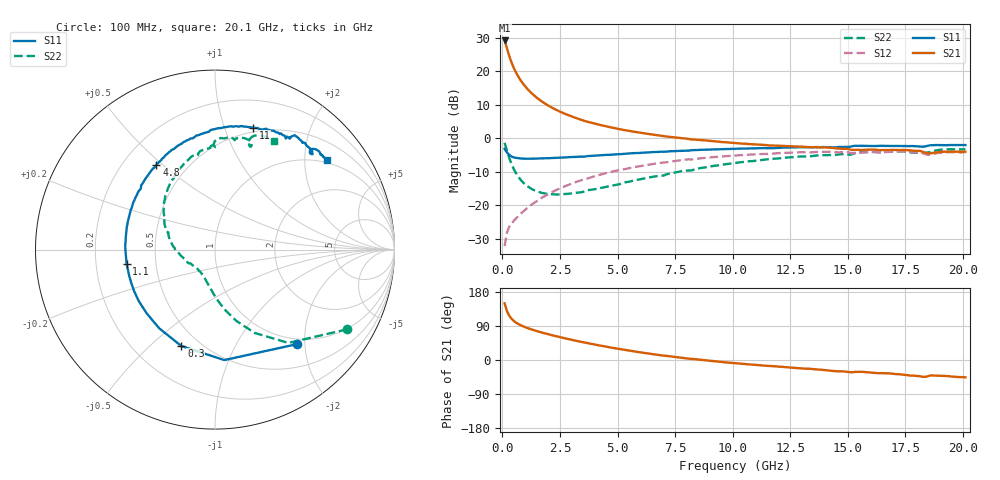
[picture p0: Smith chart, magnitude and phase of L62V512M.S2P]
!  Infineon Technologies AG
! BFR380L3 , PF131585-7, No.6, Th 09.10.01, soldered on pcb-board, measured with PP GSG850
!  Vce=2.5 V,  Ic=12.5 mA
! Common Emitter S-Parameters:  15. November 2001
#  GHz  S  MA  R  50
! f  S11  S21  S12  S22
! GHz  Mag  Ang  Mag  Ang  Mag  Ang  Mag  Ang
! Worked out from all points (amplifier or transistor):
!   201 points, 100 MHz to 20.1 GHz, reference 50 ohm
!   highest |S21| = 29.3 dB at 100 MHz (marker M1)
!   |S21| within 3 dB of that: start of sweep to 228.5 MHz
!   unconditionally stable (mu >= 1): 1.666 GHz to 4.494 GHz
!   at 3.4 GHz: K = 1.02, MAG = 8.1 dB, |S12| = -12.5 dB
!   at 10.1 GHz: K = 0.95, MSG = 1.9 dB, |S12| = -5.1 dB
!   at 20.1 GHz: K = 0.99, MSG = 0.1 dB, |S12| = -4.1 dB
!   S11 on the Smith chart (normalised r, x): 100 MHz: 0.90, -1.85; 300 MHz: 0.40, -0.63; 1.1 GHz: 0.34, -0.07; 4.8 GHz: 0.34, +0.48; 11 GHz: 0.45, +1.25; 20.1 GHz: 0.94, +2.55
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0.1  0.6979 -49.0  29.06 149.5  0.0246 66.6  0.8606 -31.1
0.2  0.6177 -85.2  22.16 129.2  0.03908 56.1  0.6614 -51.8
0.3  0.569 -109.2  17.08 117.0  0.04794 51.5  0.5135 -64.6
0.4  0.5376 -125.3  13.65 108.8  0.05358 50.3  0.4148 -73.3
0.5  0.5205 -137.0  11.28 103.0  0.05888 50.8  0.348 -79.7
0.6  0.5126 -145.8  9.578 98.6  0.06425 51.7  0.3011 -84.8
0.7  0.5067 -152.7  8.327 94.9  0.06961 52.8  0.2664 -89.1
0.8  0.5021 -158.4  7.343 91.7  0.07494 54.2  0.2403 -92.9
0.9  0.4997 -163.2  6.573 89.0  0.0807 55.2  0.2201 -96.2
1.1  0.4988 -171.0  5.439 84.2  0.09226 56.9  0.1925 -102.5
1.3  0.4979 -177.6  4.638 80.0  0.1041 58.0  0.174 -107.9
1.5  0.5006 177.2  4.049 76.3  0.1162 58.7  0.162 -113.0
2  0.507 165.9  3.087 67.9  0.1477 59.0  0.1481 -124.3
2.7  0.5195 153.2  2.345 57.5  0.1919 57.3  0.1478 -138.7
3.5  0.5344 141.1  1.86 46.9  0.2427 53.8  0.159 -151.3
4.8  0.5746 124.6  1.442 32.0  0.3208 46.5  0.1984 -172.6
6.8  0.6299 103.4  1.105 13.1  0.4289 33.4  0.2756 160.8
10.1  0.7027 78.2  0.8523 -8.5  0.5551 11.9  0.4299 127.6
11  0.712 72.8  0.813 -12.9  0.5803 6.2  0.4642 119.3
13.5  0.7385 60.6  0.7423 -24.1  0.624 -8.9  0.5478 99.4
16.8  0.7719 48.4  0.6733 -35.3  0.6303 -25.0  0.6361 77.9
20.1  0.7963 38.6  0.635 -45.8  0.6229 -38.7  0.6907 61.5
